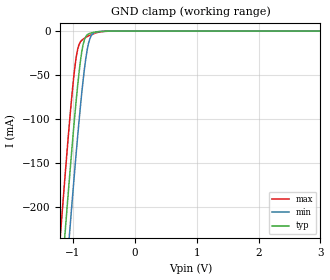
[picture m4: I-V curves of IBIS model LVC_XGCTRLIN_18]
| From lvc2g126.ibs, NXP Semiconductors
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|   Model LVC_XGCTRLIN_18
[Model]   LVC_XGCTRLIN_18
Model_type   Input
Vinl =   0.63V
Vinh =   1.17V
C_comp   3.0387pF   2.3478pF   3.8465pF
|Ambient temperature:   25   85   -40
[Temperature Range]   25   85   -40
[Voltage Range]   1.80V   1.65V   1.95V
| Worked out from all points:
|   GND clamp passes 1 mA (typ) near -0.62 V on its own axis
|Process Range   nominal   slow   fast
[GND_clamp]
| voltage   I(typ)   I(min)   I(max)
-5.5V     -4.528A    -4.585A    -4.471A
-1.208V   -305.5mA   -370.9mA   -239.5mA
-1.186V   -285.2mA   -350.6mA   -219.4mA
-1.12V    -225.4mA   -290.5mA   -160.2mA
-1.054V   -167.3mA   -231.6mA   -104mA
-988mV    -112mA     -174.4mA   -54.21mA
-944mV    -77.83mA   -137.8mA   -29.07mA
-856mV    -23.75mA   -70.75mA   -10.5mA
-768mV    -4.272mA   -21.32mA   -6.327mA
-702mV    -2.021mA   -5.071mA   -4.042mA
-400mV    -70.93uA   -77.02uA   -53.98uA
5.5V      0A         0A         0A
